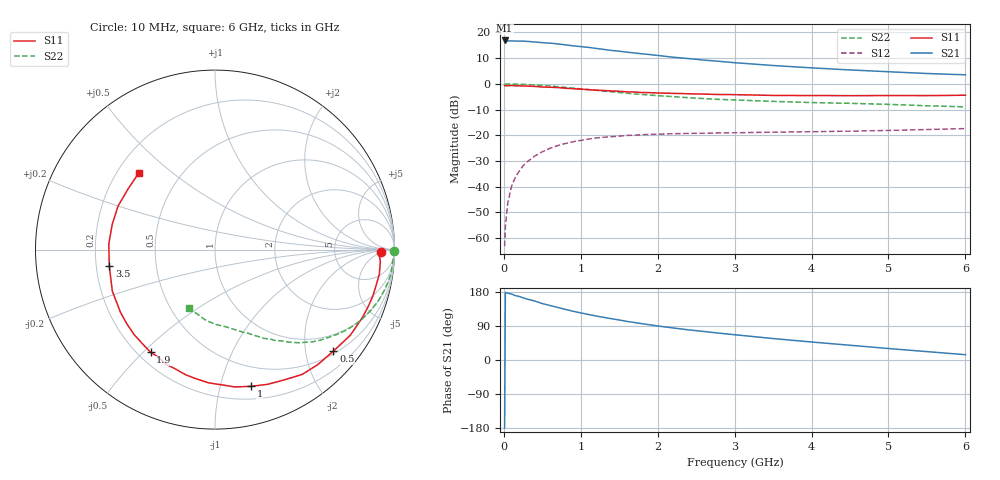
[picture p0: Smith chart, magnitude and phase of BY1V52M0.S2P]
! SIEMENS Small Signal Semiconductors
! BFY420
! Si NPN RF SIEGET Grounded Emitter Transistor in MICRO-X
! VCE = 1.5 V  IC = 2 mA
! Common Emitter S-Parameters:  October  1996
# GHz  S  MA  R  50
!  f  S11  S21  S12  S22
! GHz  MAG  ANG  MAG  ANG  MAG  ANG  MAG  ANG
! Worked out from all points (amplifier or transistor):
!   36 points, 10 MHz to 6 GHz, reference 50 ohm
!   highest |S21| = 16.9 dB at 10 MHz (marker M1)
!   |S21| within 3 dB of that: start of sweep to 1.177 GHz
!   unconditionally stable (mu >= 1): 3.979 GHz to end of sweep
!   at 250 MHz: K = 0.06, MSG = 24.2 dB, |S12| = -31.8 dB
!   at 1.4 GHz: K = 0.30, MSG = 16.8 dB, |S12| = -20.5 dB
!   at 6 GHz: K = 1.26, MAG = 7.4 dB, |S12| = -17.4 dB
!   S11 on the Smith chart (normalised r, x): 10 MHz: 25, -5; 500 MHz: 0.56, -2.60; 1 GHz: 0.31, -1.25; 1.9 GHz: 0.25, -0.53; 3.5 GHz: 0.25, -0.07; 6 GHz: 0.29, +0.38
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0.01  0.9255 -0.9  6.979 -179.5  0.0007 90.1  0.9975 -0.5
0.02  0.915 -1.7  6.919 178.4  0.0017 89.6  0.9905 -0.8
0.05  0.9237 -4.1  6.822 176.3  0.0047 89.9  0.995 -2.2
0.1  0.9258 -8.5  6.853 174.1  0.0102 86.3  0.9918 -4.5
0.15  0.9196 -12.4  6.783 169.9  0.0153 81.5  0.9896 -6.7
0.2  0.9168 -16.5  6.768 167.6  0.0201 80.2  0.9865 -8.7
0.25  0.9102 -20.5  6.772 164.1  0.0256 77.1  0.9794 -11.0
0.4  0.8924 -32.3  6.532 155.7  0.0394 71.1  0.954 -17.3
0.5  0.8689 -40.6  6.324 148.9  0.0478 66.9  0.9328 -21.2
0.7  0.8483 -55.1  5.983 138.7  0.0631 58.5  0.8824 -28.6
0.8  0.8212 -62.3  5.732 133.5  0.0694 54.1  0.8534 -32.0
1  0.7878 -75.3  5.296 124.3  0.0796 47.7  0.799 -37.8
1.1  0.773 -81.8  5.12 120.1  0.0844 44.8  0.7739 -40.7
1.4  0.7277 -98.1  4.455 108.9  0.0941 37.1  0.703 -47.6
1.6  0.6997 -108.8  4.132 101.8  0.0994 32.8  0.6572 -51.6
1.9  0.6752 -122.1  3.709 92.9  0.1041 27.7  0.6058 -56.7
2.2  0.6541 -133.3  3.298 84.6  0.1074 23.6  0.5653 -61.1
2.8  0.6209 -152.5  2.742 70.8  0.1112 18.2  0.4986 -68.8
3.5  0.5961 -171.0  2.274 56.6  0.1151 14.2  0.457 -76.5
4.5  0.5897 166.1  1.864 38.9  0.1204 10.6  0.4182 -88.8
5.5  0.5908 144.8  1.59 22.1  0.1295 8.5  0.3751 -104.3
6  0.6017 135.1  1.499 14.0  0.1353 7.4  0.3575 -113.5
